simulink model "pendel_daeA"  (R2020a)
settings: Solver=ode45  StartTime=0.0  StopTime=10  MaxStep=0.01  RelTol=1e-5  EnableMultiTasking=on
InitFcn:
  | g = 9.81;

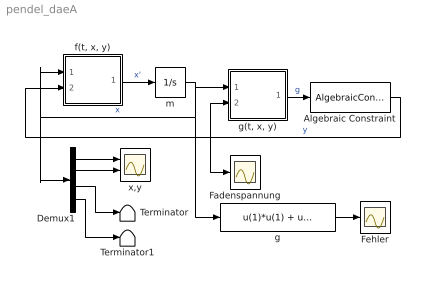
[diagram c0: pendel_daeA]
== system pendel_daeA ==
  Algebraic Constraint : AlgebraicConstraint
  Demux1 : Demux
  Fadenspannung : Scope
  Fehler : Scope
  Terminator : Terminator
  Terminator1 : Terminator
  "f(t, x, y)" : Subsystem
  g : Fcn  Expr=u(1)*u(1) + u(2)*u(2) - 1
  "g(t, x, y)" : Subsystem
  m : Integrator  InitialCondition=[1;0;0;0]
  x,y : Scope  NumInputPorts=2
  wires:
  "g(t, x, y)"/1(g) -> Algebraic Constraint/1  "g"
  Algebraic Constraint/1 -> "g(t, x, y)"/2(y), "f(t, x, y)"/2(y), Fadenspannung/1  "y"
  m/1 -> "g(t, x, y)"/1(x), "f(t, x, y)"/1(x), Demux1/1, g/1  "x"
  "f(t, x, y)"/1(f) -> m/1  "x'"
  Demux1/1 -> x,y/1
  Demux1/2 -> x,y/2
  Demux1/3 -> Terminator/1
  Demux1/4 -> Terminator1/1
  g/1 -> Fehler/1

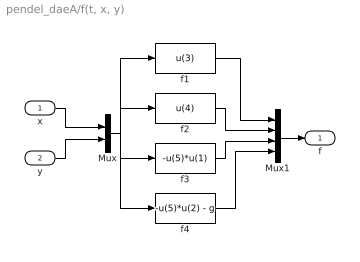
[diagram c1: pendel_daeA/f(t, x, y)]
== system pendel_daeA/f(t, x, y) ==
  x : Inport
  y : Inport  Port=2
  Mux : Mux  Inputs=2
  Mux1 : Mux
  f1 : Fcn  Expr=u(3)
  f2 : Fcn  Expr=u(4)
  f3 : Fcn  Expr=-u(5)*u(1)
  f4 : Fcn  Expr=-u(5)*u(2) - g
  f : Outport
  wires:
  x/1 -> Mux/1
  y/1 -> Mux/2
  Mux/1 -> f1/1, f2/1, f4/1, f3/1
  Mux1/1 -> f/1
  f2/1 -> Mux1/2
  f1/1 -> Mux1/1
  f3/1 -> Mux1/3
  f4/1 -> Mux1/4

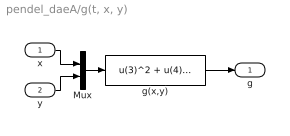
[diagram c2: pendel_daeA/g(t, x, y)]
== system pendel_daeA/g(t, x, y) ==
  x : Inport
  y : Inport  Port=2
  Mux : Mux  Inputs=2
  g(x,y) : Fcn  Expr=u(3)^2 + u(4)^2 - u(5)*(u(1)^2 + u(2)^2) - g*u(2)
  g : Outport
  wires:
  x/1 -> Mux/1
  y/1 -> Mux/2
  Mux/1 -> g(x,y)/1
  g(x,y)/1 -> g/1
